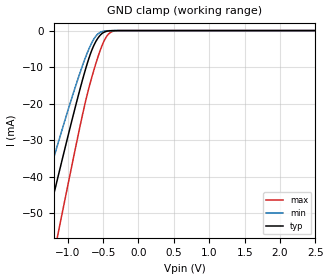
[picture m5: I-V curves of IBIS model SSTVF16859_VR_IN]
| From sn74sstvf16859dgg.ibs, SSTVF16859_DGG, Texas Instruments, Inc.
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[Model]   SSTVF16859_VR_IN
Model_type  Input
Vinl=0.7
Vinh=1.7
| variable   typ   min   max
C_comp   6.16pF   3.26pF   8.02pF
[Temperature Range]   40   85   0
| Ambient temperature   25   70   0
[Voltage range]   2.5   2.3   2.7
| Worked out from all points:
|   GND clamp passes 1 mA (typ) near -0.53 V on its own axis
[GND Clamp]
| SSTVF16859_VR_IN
|   Voltage   I(typ)   I(min)   I(max)
-2.5V     -152.2mA   -125.5mA   -186.3mA
-1.53V    -71.94mA   -57.31mA   -93.53mA
-1.48V    -67.84mA   -53.88mA   -88.71mA
-1.34V    -56.4mA    -44.37mA   -75.22mA
-1.295V   -52.75mA   -41.34mA   -70.89mA
-1.135V   -39.86mA   -30.74mA   -55.48mA
-740mV    -10.06mA   -6.918mA   -18.72mA
-635mV    -4.259mA   -2.472mA   -11.14mA
-540mV    -1.259mA   -482.8uA   -5.385mA
-435mV    -137.6uA   -41.26uA   -1.21mA
-310mV    -3.576uA   -1.314uA   -44.84uA
2.5V      604.9pA    434.8pA    6.022nA
